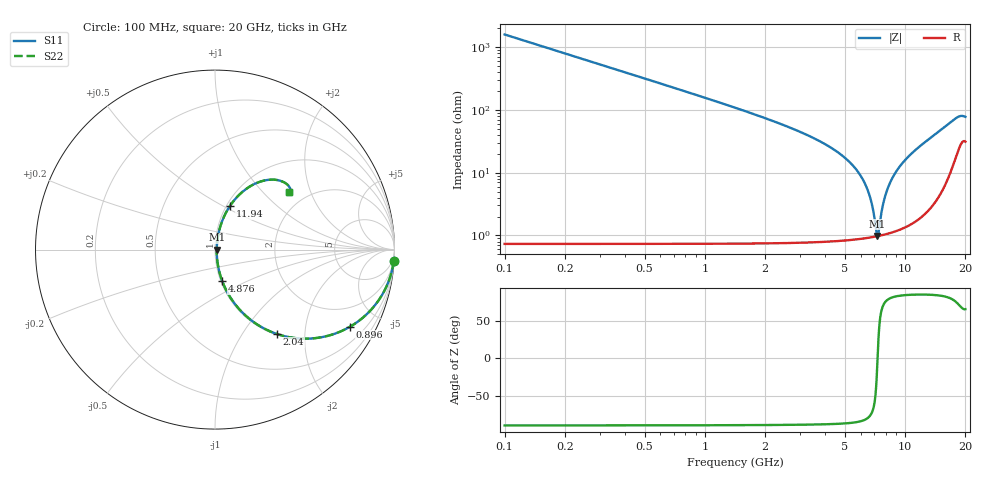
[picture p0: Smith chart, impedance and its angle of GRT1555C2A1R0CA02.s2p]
!Murata Part Number: GRT1555C2A1R0CA02
!These Parameters are Measured in Series Mode Connection
!Data Generated on Jun 19, 2026
!  o--ll--o
!Port1  Port2
!  o------o
!Operation Temp=25[degC], DC Bias Voltage=0[V]
!Freq. Start=100[MHz] Stop=20[GHz] 401[Steps]
# Hz S RI R 50
!Freq.(Hz) S11(Real) S11(Imag) S21(Real) S21(Imag) S12(Real) S12(Imag) S22(Real) S22(Imag)
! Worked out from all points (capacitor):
!   401 points, 100 MHz to 20 GHz, reference 50 ohm
!   read as one part in series: C = 1 pF near 199.5 MHz
!   lowest |Z| = 982 mohm at 7.264 GHz (marker M1)
!   series resonance near 7.284 GHz, so ESL is about 480 pH
!   S11 on the Smith chart (normalised r, x): 100 MHz: 1, -32; 896 MHz: 1.01, -3.50; 2.04 GHz: 1.01, -1.44; 4.876 GHz: 1.02, -0.37; 11.94 GHz: 1.04, +0.54; 20 GHz: 1.62, +1.42
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1e8  0.996 -0.0626  0.00396 0.0626  0.00396 0.0626  0.996 -0.0626
2.99e8  0.9656 -0.1816  0.0344 0.1816  0.0344 0.1816  0.9656 -0.1816
3.985e8  0.9403 -0.236  0.0597 0.236  0.0597 0.236  0.9403 -0.236
5.975e8  0.8744 -0.33  0.1256 0.33  0.1256 0.33  0.8744 -0.33
8.96e8  0.7531 -0.4291  0.2469 0.4291  0.2469 0.4291  0.7531 -0.4291
1.3935e9  0.5484 -0.4943  0.4516 0.4943  0.4516 0.4943  0.5484 -0.4943
2.04025e9  0.3442 -0.47  0.6558 0.47  0.6558 0.47  0.3442 -0.47
3.43325e9  0.1229 -0.3178  0.8771 0.3178  0.8771 0.3178  0.1229 -0.3178
4.876e9  0.0404 -0.1759  0.9596 0.1759  0.9596 0.1759  0.0404 -0.1759
6.07e9  0.0155 -0.0814  0.9845 0.0814  0.9845 0.0814  0.0155 -0.0814
6.7665e9  0.0104 -0.0333  0.9896 0.0333  0.9896 0.0333  0.0104 -0.0333
7.264e9  0.00964 -0.00128  0.9904 0.00128  0.9904 0.00128  0.00964 -0.00128
7.3635e9  0.00974 0.00491  0.9903 -0.00491  0.9903 -0.00491  0.00974 0.00491
7.81125e9  0.0112 0.032  0.9888 -0.032  0.9888 -0.032  0.0112 0.032
8.259e9  0.014 0.058  0.986 -0.058  0.986 -0.058  0.014 0.058
9.00525e9  0.0216 0.0991  0.9784 -0.0991  0.9784 -0.0991  0.0216 0.0991
1.005e10  0.0377 0.153  0.9623 -0.153  0.9623 -0.153  0.0377 0.153
1.19405e10  0.0823 0.2416  0.9177 -0.2416  0.9177 -0.2416  0.0823 0.2416
1.338325e10  0.1312 0.3017  0.8688 -0.3017  0.8688 -0.3017  0.1312 0.3017
1.67165e10  0.3047 0.3894  0.6953 -0.3894  0.6953 -0.3894  0.3047 0.3894
1.8607e10  0.4104 0.3546  0.5896 -0.3546  0.5896 -0.3546  0.4104 0.3546
2e10  0.4107 0.3191  0.5893 -0.3191  0.5893 -0.3191  0.4107 0.3191
